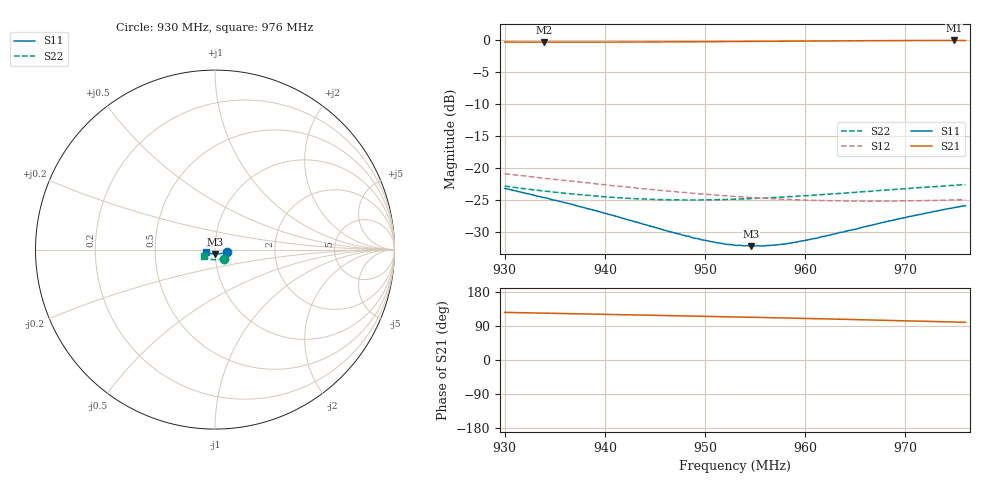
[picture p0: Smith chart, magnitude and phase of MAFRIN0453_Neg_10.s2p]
!Part Number:  MAFRIN0453
!Name:  MariaCraven
!Comments:  1
!Thu 30/Sep/2004  2:41:06 PM
!Temperature:  -10
# MHZ  S  DB  R  50
!Freq  S11(dB)  S11(ang)  S21(dB)  S21(ang)  S12(dB)  S12(ang)  S22(dB)  S22(ang)
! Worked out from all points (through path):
!   201 points, 930 MHz to 976 MHz, reference 50 ohm
!   highest |S21| = -0.06 dB at 974.85 MHz (marker M1); lowest = -0.3 dB at 933.91 MHz (marker M2)
!   lowest |S11| = -32.3 dB at 954.61 MHz (marker M3), VSWR 1.05, Z = 50.1 - j2.43 ohm
!   |S11| at or under -10 dB: start of sweep to end of sweep
!   |S22| runs from -25.1 to -22.6 dB; largest |S21 - S12| = 0.96
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930  -23.24 -13.2  -0.31 125.7  -20.93 112.2  -22.87 -44.6
933.91  -24.66 -18.3  -0.33 123.7  -21.65 113.7  -23.63 -53.1
937.82  -26.20 -24.9  -0.31 121.7  -22.28 115.9  -24.23 -62.6
941.27  -27.66 -32.0  -0.32 120.0  -22.87 118.2  -24.70 -71.6
945.41  -29.52 -43.6  -0.29 117.8  -23.52 121.6  -24.99 -82.7
948.17  -30.73 -53.6  -0.27 116.3  -23.91 124.1  -25.04 -90.1
948.4  -30.74 -54.6  -0.26 116.2  -23.95 124.5  -25.05 -90.7
948.86  -31.01 -56.6  -0.25 116.0  -24.00 125.0  -25.04 -91.9
951.16  -31.74 -67.4  -0.25 114.8  -24.29 127.3  -24.98 -98.1
953  -32.14 -77.3  -0.22 113.7  -24.49 129.4  -24.92 -102.7
953.92  -32.23 -82.7  -0.21 113.2  -24.58 130.5  -24.86 -105.0
954.15  -32.18 -83.6  -0.21 113.1  -24.62 130.8  -24.86 -105.5
954.61  -32.28 -86.3  -0.20 112.8  -24.66 131.4  -24.82 -106.8
955.99  -32.23 -94.7  -0.20 112.0  -24.79 133.0  -24.75 -110.2
958.06  -31.93 -106.9  -0.17 110.8  -24.93 135.5  -24.56 -114.8
960.82  -31.11 -121.8  -0.14 109.2  -25.11 139.0  -24.29 -121.1
961.97  -30.75 -127.3  -0.14 108.5  -25.14 140.4  -24.16 -123.4
963.35  -30.17 -133.3  -0.12 107.6  -25.19 142.1  -24.02 -126.2
963.81  -30.08 -135.0  -0.13 107.3  -25.21 142.8  -23.98 -127.3
968.41  -28.33 -150.4  -0.09 104.4  -25.22 148.2  -23.46 -136.1
974.85  -26.25 -165.7  -0.06 100.2  -25.03 155.0  -22.78 -146.8
976  -25.94 -167.8  -0.06 99.4  -24.99 156.0  -22.65 -148.6
